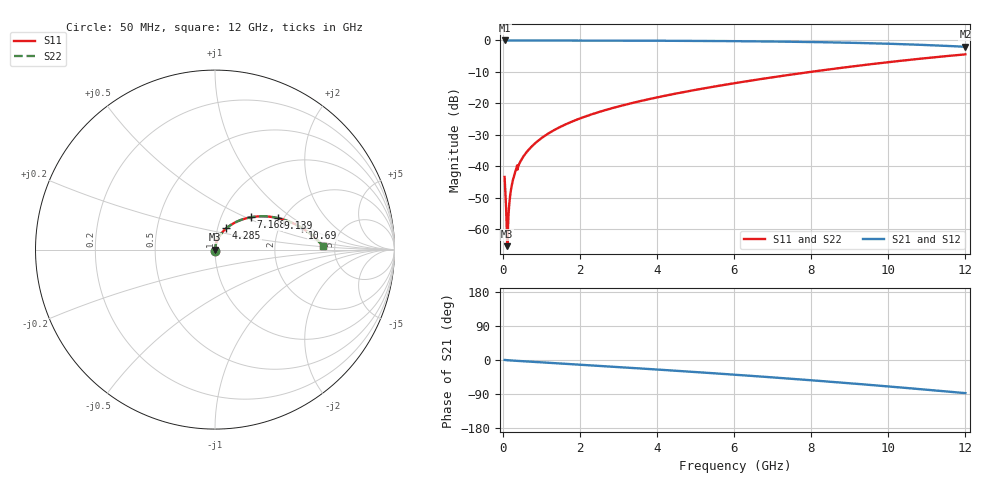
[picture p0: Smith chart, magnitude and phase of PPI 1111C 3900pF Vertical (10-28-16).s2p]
# GHz S MA R 50
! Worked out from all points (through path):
!   1601 points, 50 MHz to 12 GHz, reference 50 ohm
!   highest |S21| = 0.00 dB at 50 MHz (marker M1); lowest = -2.0 dB at 12 GHz (marker M2)
!   group delay of S21, straight-line fit = 20 ps
!   lowest |S11| = -65.4 dB at 117.2 MHz (marker M3), VSWR 1.00, Z = 50.1 - j0.0183 ohm
!   |S11| at or under -10 dB: start of sweep to 7.985 GHz
!   |S22| runs from -65.4 to -4.4 dB; largest |S21 - S12| = 0
!   S11 on the Smith chart (normalised r, x): 50 MHz: 1.00, -0.01; 4.285 GHz: 1.10, +0.27; 7.168 GHz: 1.38, +0.53; 9.139 GHz: 1.86, +0.77; 10.69 GHz: 2.70, +0.86; 12 GHz: 3.99, +0.26
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0.05  0.00676 -86.7  0.9996 0.2  0.9996 0.2  0.00676 -86.7
0.079875  0.00289 -81.5  0.9996 -0.2  0.9996 -0.2  0.00289 -81.5
0.1172187  0.000536 -19.9  0.9995 -0.5  0.9995 -0.5  0.000536 -19.9
0.1545625  0.001807 71.0  0.9994 -0.8  0.9994 -0.8  0.001807 71.0
0.1695  0.002443 75.2  0.9994 -0.9  0.9994 -0.9  0.002443 75.2
0.199375  0.003633 78.9  0.9994 -1.1  0.9994 -1.1  0.003633 78.9
0.2217813  0.00447 80.3  0.9993 -1.3  0.9993 -1.3  0.00447 80.3
0.318875  0.007845 82.4  0.9992 -1.9  0.9992 -1.9  0.007845 82.4
0.4159687  0.01044 82.7  0.999 -2.5  0.999 -2.5  0.01044 82.7
0.6026875  0.01622 82.8  0.9988 -3.7  0.9988 -3.7  0.01622 82.8
0.8491562  0.02342 81.9  0.9985 -5.2  0.9985 -5.2  0.02342 81.9
1.162844  0.03253 80.5  0.998 -7.1  0.998 -7.1  0.03253 80.5
2.044156  0.05872 75.6  0.9964 -12.6  0.9964 -12.6  0.05872 75.6
4.038312  0.1256 63.5  0.9893 -25.4  0.9893 -25.4  0.1256 63.5
4.284781  0.1349 61.9  0.988 -27.0  0.988 -27.0  0.1349 61.9
6.025  0.2097 50.3  0.9741 -38.8  0.9741 -38.8  0.2097 50.3
7.167719  0.2687 42.1  0.959 -47.1  0.959 -47.1  0.2687 42.1
8.019156  0.3183 35.6  0.9433 -53.6  0.9433 -53.6  0.3183 35.6
9.139469  0.3908 26.8  0.9152 -62.6  0.9152 -62.6  0.3908 26.8
10.01331  0.4522 19.5  0.8861 -69.9  0.8861 -69.9  0.4522 19.5
10.6855  0.5017 13.7  0.8589 -75.7  0.8589 -75.7  0.5017 13.7
12  0.6007 2.0  0.7925 -87.4  0.7925 -87.4  0.6007 2.0
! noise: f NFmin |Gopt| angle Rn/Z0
0.05  0.0004128  0.8784  0.2308  0.0007345
1.372  0.004376  0.7136  6.104  0.003006
2.701  0.007265  0.6711  11.85  0.004207
4.031  0.009909  0.649  17.42  0.005242
5.36  0.0125  0.6381  22.82  0.006272
6.682  0.01513  0.6353  28  0.007378
8.012  0.01793  0.639  33.03  0.008653
9.341  0.02099  0.6482  37.88  0.01018
10.67  0.0244  0.6623  42.58  0.01208
12  0.02833  0.6808  47.15  0.01453
